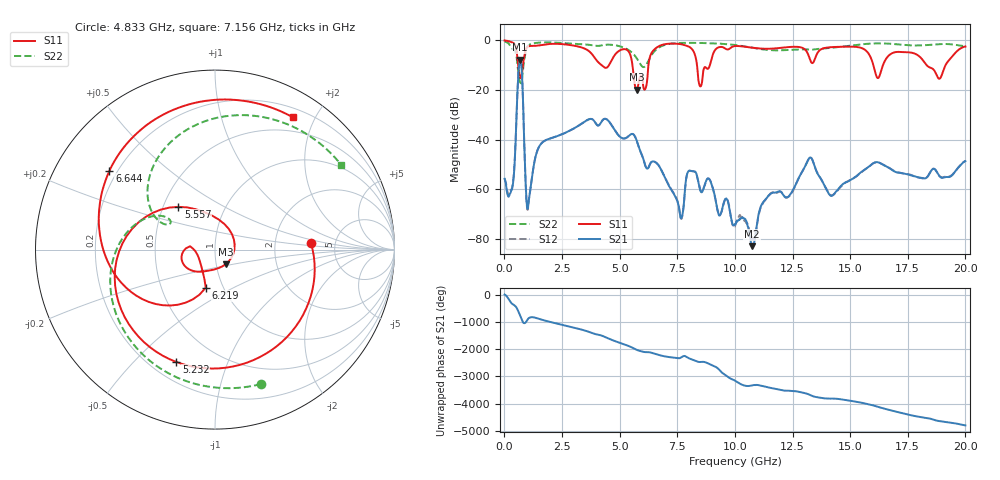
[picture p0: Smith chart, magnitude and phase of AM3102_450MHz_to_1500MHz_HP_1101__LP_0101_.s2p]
!Agilent Technologies,E8364B,MY43040894,A.07.50.67
!Agilent E8364B: A.07.50.67
!Date: Thursday, January 11, 2018 06:38:31
!Correction: S11(Full 2 Port(1,2))
!S21(Full 2 Port(1,2))
!S12(Full 2 Port(1,2))
!S22(Full 2 Port(1,2))
!S2P File: Measurements: S11, S21, S12, S22:
# Hz S  dB  R 50
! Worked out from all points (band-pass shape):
!   1601 points, 10 MHz to 20 GHz, reference 50 ohm
!   highest |S21| = -7.84 dB at 684.7 MHz (marker M1); lowest = -82.9 dB at 10.74 GHz (marker M2)
!   |S21| within 3 dB of the highest: 630.9 MHz to 744.1 MHz (113.3 MHz wide, 16.5 % of centre)
!   lowest |S11| = -19.9 dB at 5.745 GHz (marker M3), VSWR 1.22, Z = 55.6 - j9.1 ohm
!   |S11| at or under -10 dB: 5.556 GHz to 6.249 GHz (692.7 MHz wide, 11.7 % of centre); 8.357 GHz to 8.916 GHz (558.7 MHz wide, 6.47 % of centre); 18.32 GHz to 19.14 GHz (819.8 MHz wide, 4.38 % of centre)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
!   |S22| runs from -17.3 to -0.4 dB; largest |S21 - S12| = 0.0037
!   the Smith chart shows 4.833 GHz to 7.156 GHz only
!   S11 on the Smith chart (normalised r, x): 4.833 GHz: 3.27, +0.31; 5.232 GHz: 0.30, -0.67; 5.557 GHz: 0.60, +0.32; 6.219 GHz: 0.83, -0.37; 6.644 GHz: 0.17, +0.32; 7.156 GHz: 0.31, +1.71
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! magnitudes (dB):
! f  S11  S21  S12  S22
! 10 MHz  -0.1  -55.8  -55.6  -0.4
! 347.3 MHz  -0.9  -59.2  -58.8  -3.4
! 684.7 MHz  -14.8  -7.8  -7.9  -16.9
! 1.034 GHz  -2.5  -66.5  -67.0  -2.1
! 1.559 GHz  -2.0  -42.1  -42.0  -0.9
! 3.346 GHz  -2.9  -33.6  -33.6  -1.6
! 4.833 GHz  -5.4  -36.8  -36.8  -2.0
! 5.232 GHz  -3.6  -39.5  -39.5  -3.1
! 5.557 GHz  -10.1  -37.7  -37.7  -5.1
! 5.745 GHz  -19.9  -40.5  -40.5  -7.3
! 6.219 GHz  -13.2  -51.6  -51.6  -8.8
! 6.644 GHz  -2.7  -49.8  -49.8  -3.3
! 6.682 GHz  -2.5  -50.3  -50.2  -3.0
! 7.156 GHz  -1.4  -58.9  -58.7  -1.4
! 8.493 GHz  -18.5  -60.3  -60.1  -1.1
! 10.01 GHz  -2.3  -74.2  -75.0  -1.9
! 10.74 GHz  -3.0  -82.9  -79.8  -3.0
! 13.34 GHz  -9.1  -47.8  -47.8  -3.8
! 14.18 GHz  -2.8  -62.7  -62.4  -3.0
! 16.68 GHz  -6.1  -51.3  -51.3  -1.3
! 18.86 GHz  -15.5  -54.6  -54.4  -1.6
! 20 GHz  -2.5  -48.7  -48.6  -2.4
